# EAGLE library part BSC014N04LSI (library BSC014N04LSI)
MOSFET N-Ch 40V 100A TDSON-8 FL OptiMOS Source: Datasheet
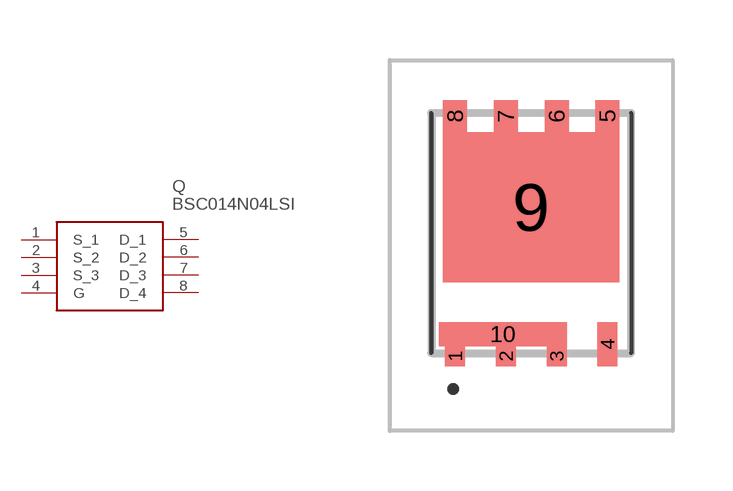
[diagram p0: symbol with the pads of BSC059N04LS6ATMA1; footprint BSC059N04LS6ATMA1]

Designator prefix Q

## BSC014N04LSI (Description: MOSFET N-Ch 40V 100A TDSON-8 FL OptiMOS; Height: mm; Manufacturer_Name: Infineon; Manufacturer_Part_Number: BSC014N04LSI; Mouser_Part_Number: 726-BSC014N04LSI; Mouser_Price-Stock: https://www.mouser.co.uk/ProductDetail/Infineon-Technologies/BSC014N04LSI?qs=EUA%2Fg8wssK0pTQXNTFzAjQ%3D%3D)  [BSC059N04LS6ATMA1]
1  S_1
2  S_2
3  S_3
4  G
5  D_1
6  D_2
7  D_3
8  D_4

## Footprint BSC059N04LS6ATMA1 (pad centres in mm)
TDSON-8 FL
smd 0.5 x 0.5: 1 -1.905,-2.764; 2 -0.635,-2.764; 3 0.635,-2.764
smd 0.5 x 1.1: 4 1.905,-2.464
smd 0.6 x 0.8: 5 1.905,3.236; 6 0.635,3.236; 7 -0.635,3.236; 8 -1.905,3.236
smd 4.41 x 3.75: 9 0,0.961
smd 3.2 x 0.6: 10 -0.715,-2.214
